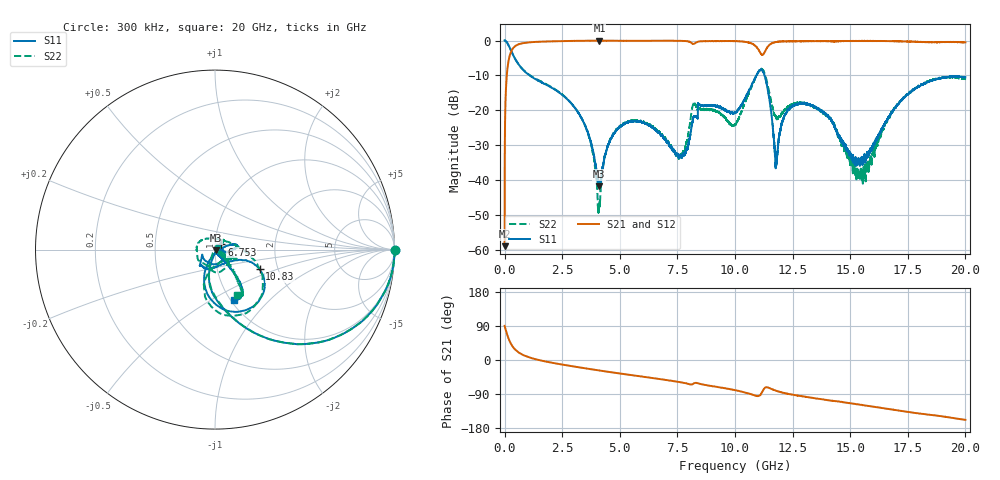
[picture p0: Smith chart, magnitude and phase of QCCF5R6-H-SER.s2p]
!QCCF5R6
!Johanson Technology Inc.
!www.johansontechnology.com
!Test Board Conditions:
!Substrate Type  RO4350B
!Substrate Thickness  10 mil
!Substrate Dk  3.66
!TL Type: GCPW
!TL Trace Width  21 mil
!TL Gap  20 mil
!Electrode orientation  Horizontal
!DUT TOPOLOGY	SERIES
!Mounting Pad LxW  16x21 mil
# MHz S  dB  R 50
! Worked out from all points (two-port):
!   20001 points, 300 kHz to 20 GHz, reference 50 ohm
!   highest |S21| = -0.02 dB at 4.114 GHz (marker M1); lowest = -59.0 dB at 300 kHz (marker M2)
!   |S21| within 3 dB of the highest: 292.8 MHz to 11.06 GHz (10.76 GHz wide, 190 % of centre); 11.31 GHz to end of sweep
!   lowest |S11| = -41.8 dB at 4.096 GHz (marker M3), VSWR 1.02, Z = 50.7 - j0.462 ohm
!   |S11| at or under -10 dB: 1.085534 GHz to 1.087284 GHz (1.75 MHz wide, 0.161 % of centre); 1.089 GHz to 10.93 GHz (9.843 GHz wide, 164 % of centre); 11.28 GHz to end of sweep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
!   |S22| runs from -49.4 to 0.0 dB; largest |S21 - S12| = 0.027
!   S11 on the Smith chart (normalised r, x): 300 kHz: open; 6.753 GHz: 1.07, +0.06; 10.83 GHz: 1.61, -0.38; 20 GHz: 1.04, -0.64
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0.3  0.04 -0.2  -58.99 90.2  -59.31 90.9  0.03 -0.1
114.298  -0.64 -23.2  -8.59 66.5  -8.61 66.7  -0.64 -23.3
334.295  -3.66 -52.5  -2.53 36.9  -2.51 37.0  -3.68 -52.6
1053.284  -9.83 -82.9  -0.51 7.3  -0.51 7.2  -9.74 -81.9
3334.25  -22.19 -106.2  -0.06 -20.4  -0.05 -20.3  -22.24 -110.8
4096.239  -41.77 -34.0  -0.03 -27.5  -0.03 -27.5  -47.77 145.2
4114.238  -41.42 -21.7  -0.02 -27.6  -0.03 -27.7  -47.65 124.7
4399.234  -32.07 40.5  -0.03 -30.3  -0.03 -30.3  -32.14 67.2
4903.226  -25.37 48.6  -0.05 -34.7  -0.05 -34.8  -25.15 58.1
6667.2  -26.34 42.0  -0.06 -49.8  -0.06 -49.8  -25.97 40.5
6753.199  -26.86 38.9  -0.05 -50.6  -0.05 -50.6  -26.64 41.3
7639.185  -32.87 51.7  -0.09 -58.8  -0.10 -58.8  -32.82 7.7
8227.177  -21.81 -97.1  -0.92 -61.4  -0.93 -61.4  -17.79 -82.5
10000.15  -20.61 -57.4  -0.15 -79.7  -0.17 -79.3  -24.21 65.8
10829.14  -11.32 -23.7  -1.22 -93.1  -1.14 -93.0  -11.59 -22.5
11293.13  -10.25 -88.7  -3.24 -73.7  -3.27 -74.0  -9.59 -91.1
11789.12  -35.42 -35.4  -0.43 -81.3  -0.45 -81.4  -22.01 -71.9
12252.12  -20.41 16.1  -0.21 -88.7  -0.23 -88.5  -19.38 -29.4
13334.1  -18.73 5.6  -0.16 -99.6  -0.18 -99.6  -18.76 -24.1
15466.07  -34.38 -56.0  -0.11 -118.2  -0.09 -118.3  -37.18 -24.2
16667.05  -21.96 -51.9  -0.12 -129.3  -0.10 -129.7  -21.83 -40.9
20000  -10.52 -68.8  -0.49 -157.9  -0.37 -156.8  -11.01 -63.9
